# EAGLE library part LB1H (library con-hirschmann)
Female RF CONNECTOR with switch, horizontal
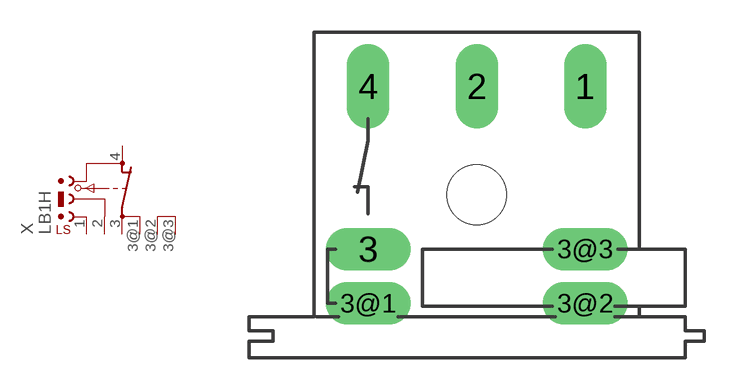
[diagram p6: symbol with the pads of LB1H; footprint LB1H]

Designator prefix X

## LB1H (OC_FARNELL: unknown; OC_NEWARK: unknown)  [LB1H]
1  1  pas
2  2  pas
3  3  pas
3@1  3A  pas
3@2  3B  pas
3@3  3C  pas
4  4  pas

## Footprint LB1H (pad centres in mm)
Female RF CONNECTOR with switch horizontal
drill 1.321 long: 1 5.08,5.08; 2 0,5.08; 3 -5.08,-2.54; 3@1 -5.08,-5.08; 3@2 5.08,-5.08; 3@3 5.08,-2.54; 4 -5.08,5.08
hole 2.794 at 0,0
